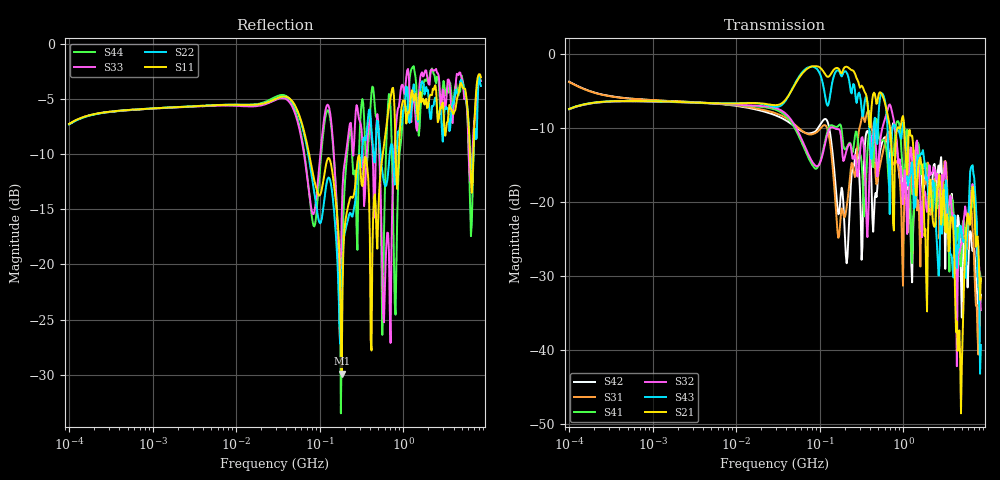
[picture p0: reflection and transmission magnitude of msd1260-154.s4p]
# MHz S MA R 50
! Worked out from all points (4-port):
!   498 points, 100 kHz to 8.5 GHz, reference 50 ohm
!   strongest paths, dB at 100 kHz, 1.698 MHz, 29.49 MHz, 500.7 MHz, 8.5 GHz:
!     S21: -7.4, -6.4, -6.9, -5.8, -30.3
!     S43: -7.4, -6.4, -7.1, -9.4, -39.3
!     S32: -7.4, -6.4, -7.3, -15.7, -34.6
!     S41: -7.4, -6.5, -7.5, -10.3, -30.7
!     S31: -3.7, -6.3, -8.0, -16.5, -32.9
!     S42: -3.7, -6.3, -8.2, -15.8, -32.5
!   lowest |S11| = -29.9 dB at 183.3 MHz (marker M1), VSWR 1.07, Z = 53.3 - j0.0537 ohm
!   |S11| at or under -10 dB: 74.8 MHz to 568.7 MHz (493.9 MHz wide, 153 % of centre); 813.6 MHz to 884.2 MHz (70.56 MHz wide, 8.31 % of centre); 6.303 GHz to 6.911 GHz (608.1 MHz wide, 9.2 % of centre)
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0.1  0.434 29.0  0.427 28.8  0.651 -19.2  0.425 -151.8
     0.427 28.8  0.4318 29.0  0.4253 -151.7  0.6522 -19.2
     0.651 -19.2  0.4253 -151.7  0.4332 29.0  0.4268 28.7
     0.425 -151.8  0.6522 -19.2  0.4268 28.7  0.4326 29.1
183.289  0.0319 -0.9  0.7429 -32.5  0.09065 -79.4  0.3082 29.8
         0.7429 -32.5  0.07545 96.6  0.2455 20.4  0.1252 -48.7
         0.09065 -79.4  0.2455 20.4  0.1634 41.0  0.7093 -37.6
         0.3082 29.8  0.1252 -48.7  0.7093 -37.6  0.04239 82.1
2260.241  0.6272 -179.6  0.07478 49.8  0.1347 138.9  0.08736 134.3
          0.07478 49.8  0.522 175.3  0.1629 142.7  0.1541 148.8
          0.1347 138.9  0.1629 142.7  0.7618 174.5  0.1401 64.6
          0.08736 134.3  0.1541 148.8  0.1401 64.6  0.7572 170.7
3488.216  0.4879 31.9  0.04642 123.9  0.07438 -28.8  0.05671 -12.8
          0.04642 123.9  0.4767 12.5  0.09494 4.1  0.08324 -15.3
          0.07438 -28.8  0.09494 4.1  0.6911 10.3  0.06458 169.3
          0.05671 -12.8  0.08324 -15.3  0.06458 169.3  0.6016 19.9
4802.421  0.6593 -86.1  0.008682 -24.6  0.04237 -92.8  0.03775 -84.6
          0.008682 -24.6  0.6753 -87.6  0.048 -59.4  0.05193 -162.2
          0.04237 -92.8  0.048 -59.4  0.7425 -90.1  0.06933 64.1
          0.03775 -84.6  0.05193 -162.2  0.06933 64.1  0.6078 -86.9
6764.496  0.2396 79.5  0.1274 25.5  0.06487 20.0  0.1111 82.8
          0.1274 25.5  0.2603 70.4  0.1328 74.4  0.04675 49.4
          0.06487 20.0  0.1328 74.4  0.3301 43.1  0.1777 44.9
          0.1111 82.8  0.04675 49.4  0.1777 44.9  0.2127 63.6
8500  0.707 -53.1  0.03047 -100.4  0.02266 -77.4  0.02921 -126.7
      0.03047 -100.4  0.6458 -42.5  0.0186 -103.9  0.02365 -97.2
      0.02266 -77.4  0.0186 -103.9  0.6792 -50.1  0.01081 -12.8
      0.02921 -126.7  0.02365 -97.2  0.01081 -12.8  0.6817 -53.1
